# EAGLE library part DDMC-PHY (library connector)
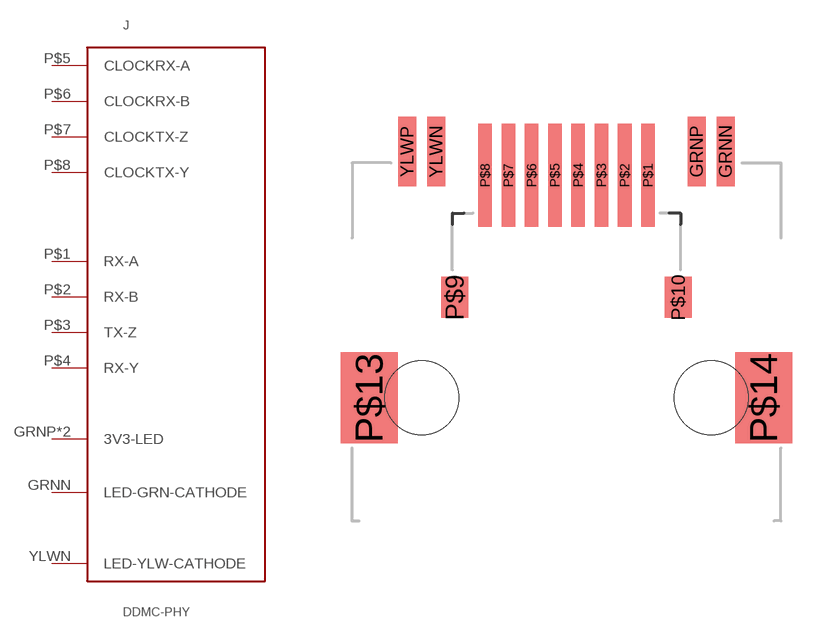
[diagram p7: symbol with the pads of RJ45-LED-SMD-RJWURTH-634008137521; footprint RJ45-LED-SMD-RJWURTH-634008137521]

Designator prefix J

## DDMC-PHYRJ45TABUPSMD  [RJ45-LED-SMD-RJWURTH-634008137521]
GRNN  LED-GRN-CATHODE
GRNP  3V3-LED
P$1  RX-A
P$2  RX-B
P$3  TX-Z
P$4  RX-Y
P$5  CLOCKRX-A
P$6  CLOCKRX-B
P$7  CLOCKTX-Z
P$8  CLOCKTX-Y
YLWN  LED-YLW-CATHODE
YLWP  3V3-LED

## Footprint RJ45-LED-SMD-RJWURTH-634008137521 (pad centres in mm)
smd 0.8 x 3.05: GRNN 6.98,10.8; GRNP 5.71,10.8; YLWN -5.71,10.8; YLWP -6.98,10.8
smd 0.6 x 4.5: P$1 3.57,9.76; P$2 2.55,9.76; P$3 1.53,9.76; P$4 0.51,9.76; P$5 -0.51,9.76; P$6 -1.53,9.76; P$7 -2.55,9.76; P$8 -3.57,9.76
smd 1.2 x 1.8: P$9 -4.9,4.4; P$10 4.9,4.4
smd 2.5 x 4: P$13 -8.65,0; P$14 8.65,0
hole 3.25 at -6.35,0
hole 3.25 at 6.35,0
